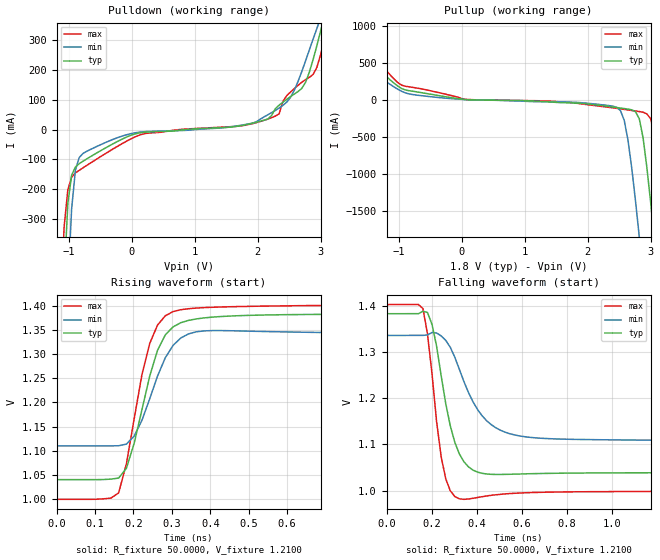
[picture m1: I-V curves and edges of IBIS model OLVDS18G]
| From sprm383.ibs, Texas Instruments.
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|   Model OLVDS18G
[Model]   OLVDS18G
Model_type   Output
Polarity   Non-Inverting
Vmeas =   1.2100V
Cref =   5.0000pF
Rref =  50.0000
Vref =   1.2100V
C_comp   1.0000pF   1.0000pF   1.0000pF
[Temperature Range]   25.0000   0.1250k   -40.0000
[Pullup Reference]   1.8000V   1.6200V   1.9500V
[Pulldown Reference]   0.000V   0.000V   0.000V
[POWER Clamp Reference]   1.8000V   1.6200V   1.9500V
[GND Clamp Reference]   0.000V   0.000V   0.000V
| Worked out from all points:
|   slope of the pulldown table from 0 to 0.27 V, typ, clamps not added: 26.9 ohm
|   slope of the pullup table from 0 to 0.27 V, typ, clamps not added: 23.1 ohm
|   rising waveform, R_fixture 50.0000, V_fixture 1.2100: 20-80 % time 67.6ps typ, 65.5ps min, 59ps max; typ from 1.04 V to 1.38 V
|   falling waveform, R_fixture 50.0000, V_fixture 1.2100: 20-80 % time 79.7ps typ, 139ps min, 55ps max; typ from 1.38 V to 1.04 V
[Pulldown]
| voltage   I(typ)   I(min)   I(max)
-1.8V     -6.631A    -6.906A    -6.482A
-1.14V    -900.4mA   -1.359A    -648.8mA
-1.08V    -503.6mA   -913.1mA   -329mA
-1.02V    -247.9mA   -534.3mA   -202mA
-900mV    -125.6mA   -136.2mA   -145.2mA
-780mV    -105.9mA   -79.86mA   -128.2mA
180mV     -8.811mA   -6.838mA   -14.19mA
2.16V     35.64mA    50.35mA    35.93mA
2.52V     111mA      108.3mA    126.6mA
2.94V     282.4mA    340.1mA    209.5mA
3.12V     434mA      448.9mA    364.9mA
3.6V      824.5mA    765.5mA    838.5mA
[Pullup]
| voltage   I(typ)   I(min)   I(max)
-1.8V     783.3mA    610.9mA    970mA
-960mV    153.3mA    115.9mA    198.9mA
60mV      4.024mA    2.149mA    7.051mA
2.46V     -102.7mA   -99.69mA   -113.9mA
2.58V     -116.5mA   -274mA     -127.9mA
2.64V     -123.8mA   -541.3mA   -135mA
2.82V     -254.6mA   -1.846A    -157mA
2.94V     -906.5mA   -2.858A    -188mA
3V        -1.375A    -3.364A    -252.8mA
3.06V     -1.879A    -3.87A     -471.7mA
3.24V     -3.463A    -5.39A     -1.87A
3.48V     -5.58A     -7.416A    -4.036A
[Ramp]
| variable   typ   min   max
dV/dt_r   0.5542/0.2033n   0.4048/0.2321n   0.6461/0.1633n
dV/dt_f   44.8237m/39.2456p   34.1854m/68.4096p   76.8482m/26.6063p
R_load = 50.0000
[Rising Waveform]
R_fixture = 50.0000
V_fixture = 1.2100
V_fixture_min = 1.2200
V_fixture_max = 1.2000
| time   V(typ)   V(min)   V(max)
0s        1.04V      1.11V      999.1mV
161.6ps   1.043V     1.11V      1.012V
181.8ps   1.064V     1.114V     1.073V
202ps     1.115V     1.13V      1.166V
222.2ps   1.185V     1.163V     1.258V
242.4ps   1.255V     1.208V     1.322V
262.6ps   1.308V     1.254V     1.36V
303ps     1.357V     1.318V     1.388V
383.8ps   1.375V     1.348V     1.397V
10ns      1.383V     1.339V     1.403V
[Falling Waveform]
R_fixture = 50.0000
V_fixture = 1.2100
V_fixture_min = 1.2200
V_fixture_max = 1.2000
| time   V(typ)   V(min)   V(max)
0s        1.382V     1.335V     1.402V
161.6ps   1.388V     1.336V     1.394V
181.8ps   1.385V     1.337V     1.339V
202ps     1.359V     1.342V     1.252V
242.4ps   1.249V     1.335V     1.073V
282.8ps   1.14V      1.31V      1V
323.2ps   1.079V     1.262V     982.6mV
424.2ps   1.038V     1.162V     987.2mV
585.9ps   1.036V     1.119V     995mV
2ns       1.039V     1.108V     998.7mV
